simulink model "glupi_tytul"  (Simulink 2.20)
settings: Solver=ode45  StartTime=0.0  StopTime=20.0  RelTol=1e-3  AbsTol=1e-6

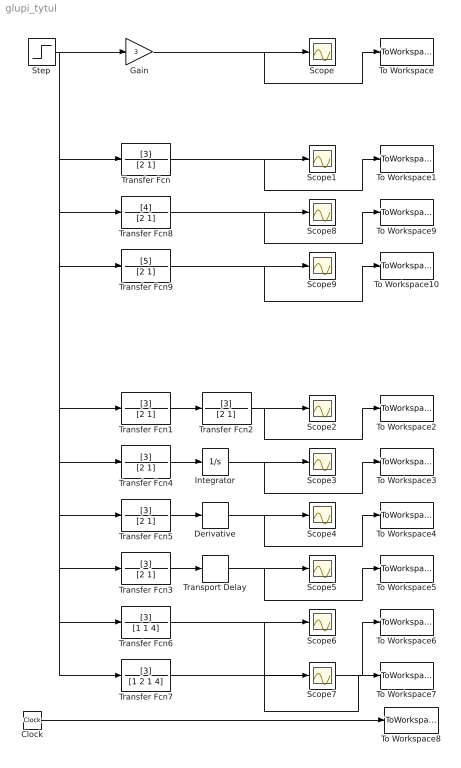
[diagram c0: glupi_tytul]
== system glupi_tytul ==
  Clock : Clock
  Derivative : Derivative
  Gain : Gain  Gain=3
  Integrator : Integrator  ExternalReset=none  InitialConditionSource=internal  InitialCondition=0  LimitOutput=off  UpperSaturationLimit=inf  LowerSaturationLimit=-inf  ShowSaturationPort=off  ShowStatePort=off  AbsoluteTolerance=auto
  Scope{,1..9} (10 alike) : Scope
  Step : Step  Time=0  Before=0  After=1
  To Workspace : ToWorkspace  VariableName=wyk_0  SampleTime=-1
  To Workspace1 : ToWorkspace  VariableName=wyk_1a  SampleTime=-1
  To Workspace10 : ToWorkspace  VariableName=wyk_1c  SampleTime=-1
  To Workspace2 : ToWorkspace  VariableName=wyk_2  SampleTime=-1
  To Workspace3 : ToWorkspace  VariableName=wyk_3  SampleTime=-1
  To Workspace4 : ToWorkspace  VariableName=wyk_4  SampleTime=-1
  To Workspace5 : ToWorkspace  VariableName=wyk_5  SampleTime=-1
  To Workspace6 : ToWorkspace  VariableName=wyk_6  SampleTime=-1
  To Workspace7 : ToWorkspace  VariableName=wyk_7  SampleTime=-1
  To Workspace8 : ToWorkspace  VariableName=t  SampleTime=-1
  To Workspace9 : ToWorkspace  VariableName=wyk_1b  SampleTime=-1
  Transfer Fcn{,1..5} (6 alike) : TransferFcn  Numerator=[3]  Denominator=[2 1]
  Transfer Fcn6 : TransferFcn  Numerator=[3]  Denominator=[1 1 4]
  Transfer Fcn7 : TransferFcn  Numerator=[3]  Denominator=[1 2 1 4]
  Transfer Fcn8 : TransferFcn  Numerator=[4]  Denominator=[2 1]
  Transfer Fcn9 : TransferFcn  Numerator=[5]  Denominator=[2 1]
  Transport Delay : TransportDelay  DelayTime=2  InitialInput=0  BufferSize=1024
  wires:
  Step/1 -> Transfer Fcn/1, Transfer Fcn8/1, Transfer Fcn1/1, Transfer Fcn4/1, Transfer Fcn5/1, Transfer Fcn3/1, Transfer Fcn6/1, Transfer Fcn7/1, Transfer Fcn9/1, Gain/1
  Gain/1 -> Scope/1, To Workspace/1
  Transfer Fcn/1 -> Scope1/1, To Workspace1/1
  Transfer Fcn8/1 -> To Workspace9/1, Scope8/1
  Transfer Fcn9/1 -> Scope9/1, To Workspace10/1
  Clock/1 -> To Workspace8/1
  Transfer Fcn1/1 -> Transfer Fcn2/1
  Transfer Fcn4/1 -> Integrator/1
  Transfer Fcn5/1 -> Derivative/1
  Transfer Fcn3/1 -> Transport Delay/1
  Transfer Fcn6/1 -> Scope6/1, To Workspace6/1
  Transport Delay/1 -> Scope5/1, To Workspace5/1
  Derivative/1 -> Scope4/1, To Workspace4/1
  Integrator/1 -> Scope3/1, To Workspace3/1
  Transfer Fcn2/1 -> Scope2/1, To Workspace2/1
  Transfer Fcn7/1 -> Scope7/1, To Workspace7/1
